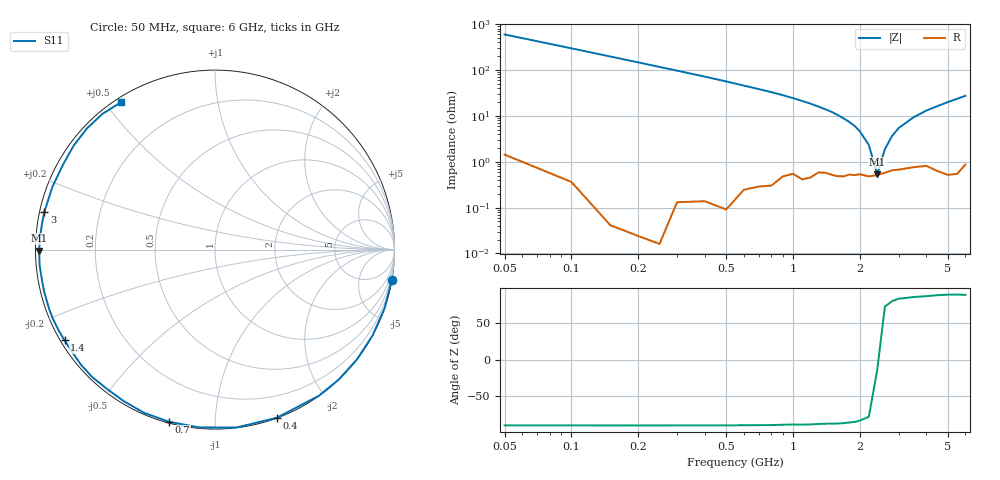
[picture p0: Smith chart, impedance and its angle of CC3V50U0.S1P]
! Infineon Technologies  Discrete & RF Semiconductors
! BBY57-02W
! Si Tuning Diode in SCD-80
! VR = 3.5 V
! S-Parameters:  June  2000
# GHz  S  MA  R  50
!  f  S11
! GHz  MAG  ANG
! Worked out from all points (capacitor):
!   34 points, 50 MHz to 6 GHz, reference 50 ohm
!   read as one part to ground: C = 5.35 pF near 50 MHz
!   lowest |Z| = 529 mohm at 2.4 GHz (marker M1)
!   series resonance near 2.414 GHz, so ESL is about 810 pH
!   S11 on the Smith chart (normalised r, x): 50 MHz: 0, -12; 400 MHz: 0.00, -1.43; 700 MHz: 0.01, -0.77; 1.4 GHz: 0.01, -0.28; 3 GHz: 0.01, +0.11; 6 GHz: 0.02, +0.55
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0.05  0.9996 -9.6
0.1  0.9996 -19.1
0.15  0.9999 -28.5
0.2  0.9999 -37.6
0.25  0.9999 -46.4
0.3  0.9989 -54.6
0.4  0.9982 -69.8
0.5  0.9984 -83.2
0.6  0.9947 -95.1
0.7  0.9928 -104.9
0.8  0.9916 -113.4
0.9  0.9856 -121.1
1  0.9825 -128.0
1.1  0.9861 -134.2
1.2  0.9842 -139.5
1.4  0.9789 -148.9
1.6  0.9817 -156.7
1.7  0.9815 -160.3
1.9  0.9802 -166.4
2.2  0.9811 -174.8
2.4  0.9797 -179.7
3  0.9738 167.7
3.5  0.9711 159.0
4  0.9701 150.8
4.5  0.9777 143.7
5  0.9823 136.5
5.5  0.9824 129.7
6  0.9738 122.6
